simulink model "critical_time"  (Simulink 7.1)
settings: Solver=ode3  StartTime=0.0  StopTime=0.3  FixedStep=1e-4  MaxStep=1e  RelTol=1e-3
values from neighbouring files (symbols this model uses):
  delta_1 = angle(EP)    [calculation.m]
  H = 3.5    [calculation.m]
  P_Peak_Fault = EP_Mag*VTH/XT_Fault,    [calculation.m]
  Pm_PU = Pm/MVA_Base    (= 1)    [calculation.m]
  Wsyn = 2*pi*60    (= 376.991118431)    [calculation.m]

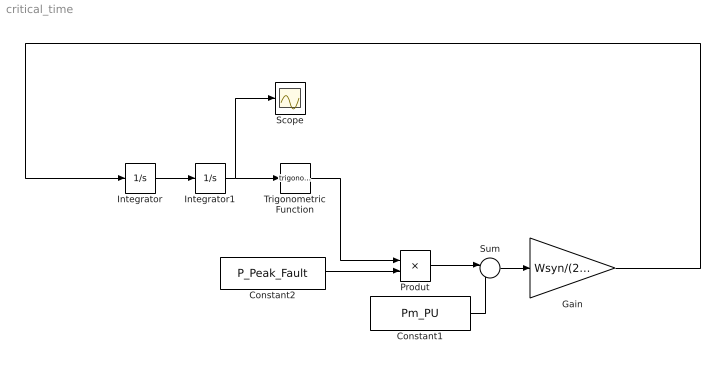
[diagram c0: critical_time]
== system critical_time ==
  Constant1 : Constant  Value=Pm_PU  OutDataType=sfix(16)  OutScaling=2^0
  Constant2 : Constant  Value=P_Peak_Fault  OutDataType=sfix(16)  OutScaling=2^0
  Gain : Gain  Gain=Wsyn/(2*H)  ParameterDataType=sfix(16)  ParameterScaling=2^0  OutDataType=sfix(16)  OutScaling=2^0
  Integrator : Integrator
  Integrator1 : Integrator  InitialCondition=delta_1
  Produt : Product  OutDataType=sfix(16)  OutScaling=2^0
  Scope : Scope
  Sum : Sum  Inputs=|-+  OutDataType=sfix(16)  OutScaling=2^0
  Trigonometric Function : Trigonometry
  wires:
  Integrator/1 -> Integrator1/1
  Integrator1/1 -> Trigonometric Function/1, Scope/1
  Trigonometric Function/1 -> Produt/1
  Constant1/1 -> Sum/2
  Produt/1 -> Sum/1
  Sum/1 -> Gain/1
  Gain/1 -> Integrator/1
  Constant2/1 -> Produt/2
